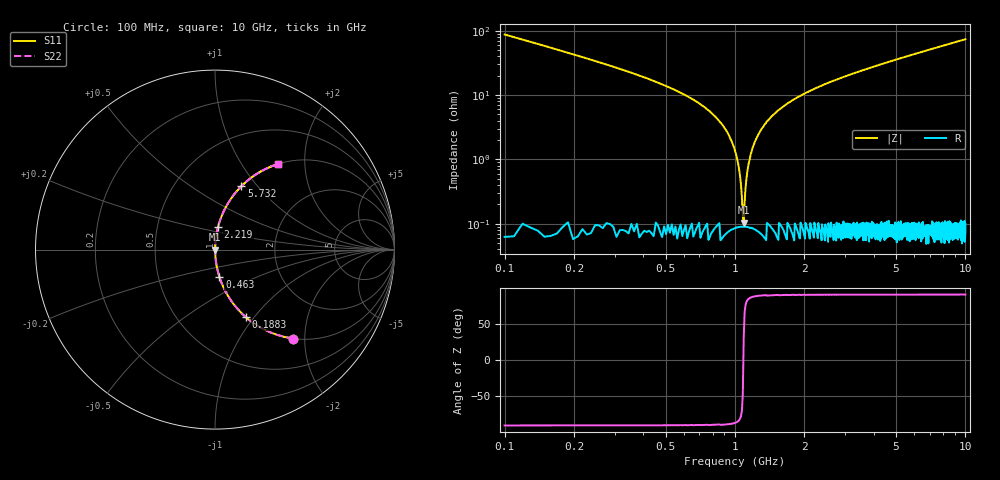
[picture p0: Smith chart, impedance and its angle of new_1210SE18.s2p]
!	AVX	Thin	Film	Operation	Date:	April 2007
!	Description:	Accu-P®	"Series,"	Thin	"Film,"	"SMD,"	RF	Capacitor
!	Part	Number:	12101J180FBT
!	100	MHz	-	5.05	GHz
!	Serial	Measurements
#	MHZ	S	MA	R	50
!	S11	S21	S12	S22
!	dB	Phase	dB	Phase	dB	Phase	dB	Phase
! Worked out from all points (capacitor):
!   1010 points, 100 MHz to 10 GHz, reference 50 ohm
!   read as one part in series: C = 18 pF near 149.1 MHz
!   lowest |Z| = 104 mohm at 1.091 GHz (marker M1)
!   series resonance near 1.088 GHz, so ESL is about 1.2 nH
!   S11 on the Smith chart (normalised r, x): 100 MHz: 1.00, -1.75; 188.3 MHz: 1.00, -0.91; 463 MHz: 1.00, -0.31; 2.219 GHz: 1.00, +0.25; 5.732 GHz: 1.00, +0.83; 10 GHz: 1.00, +1.48
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100  0.659 -48.7  0.752 41.2  0.752 41.2  0.659 -48.7
188.305  0.414 -65.4  0.909 24.5  0.909 24.5  0.414 -65.4
463.033  0.154 -80.8  0.987 8.9  0.987 8.9  0.154 -80.8
727.948  0.067 -85.5  0.997 3.8  0.997 3.8  0.067 -85.5
894.747  0.032 -86.7  0.999 1.8  0.999 1.8  0.032 -86.7
983.053  0.016 -86.3  0.999 0.9  0.999 0.9  0.016 -86.3
1012.488  0.012 -85.4  0.999 0.7  0.999 0.7  0.012 -85.4
1051.734  0.0055 -81.3  0.999 0.3  0.999 0.3  0.0055 -81.3
1090.981  0.000952 32.8  0.999 -0.0  0.999 -0.0  0.000952 32.8
1120.416  0.00491 80.3  0.999 -0.3  0.999 -0.3  0.00491 80.3
1159.663  0.01 85.0  0.999 -0.6  0.999 -0.6  0.01 85.0
1189.098  0.015 86.0  0.999 -0.8  0.999 -0.8  0.015 86.0
1297.027  0.029 86.8  0.999 -1.6  0.999 -1.6  0.029 86.8
1483.449  0.051 86.2  0.998 -2.9  0.998 -2.9  0.051 86.2
1758.176  0.081 84.8  0.996 -4.6  0.996 -4.6  0.081 84.8
2219.326  0.125 82.5  0.991 -7.2  0.991 -7.2  0.125 82.5
3406.541  0.223 76.9  0.974 -12.9  0.974 -12.9  0.223 76.9
5054.906  0.339 70.1  0.94 -19.8  0.94 -19.8  0.339 70.1
5731.913  0.382 67.5  0.924 -22.4  0.924 -22.4  0.382 67.5
6703.271  0.438 63.9  0.898 -26.0  0.898 -26.0  0.438 63.9
8351.635  0.523 58.4  0.852 -31.5  0.852 -31.5  0.523 58.4
10000  0.594 53.5  0.804 -36.4  0.804 -36.4  0.594 53.5
